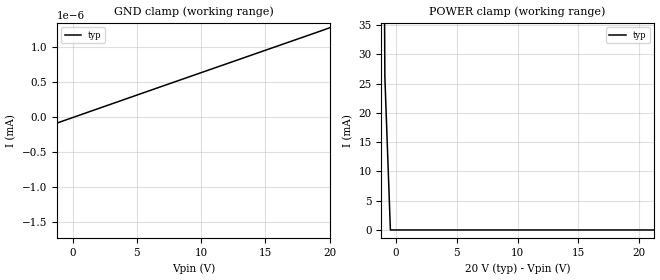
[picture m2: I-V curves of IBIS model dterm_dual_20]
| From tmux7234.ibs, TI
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| dterm_dual_20
[Model]   dterm_dual_20
Model_type   Terminator
|   typ   min   max
C_comp   1.598234e-11   NA   NA
[Voltage Range]   20   NA   NA
[Temperature Range]   27   NA   NA
[Power Clamp Reference]   20   NA   NA
[GND Clamp Reference]   0   NA   NA
[GND Clamp]
|   Voltage   I(typ)   I(min)   I(max)
-25V      -2.386A    NA         NA
-20.45V   -755.1nA   NA         NA
-20V      -1.317nA   NA         NA
-4.091V   -271.4pA   NA         NA
20V       1.28nA     NA         NA
[POWER Clamp]
|   Voltage   I(typ)   I(min)   I(max)
-5V       3.082A     NA         NA
-1.364V   208.9mA    NA         NA
-909.1mV  26.14mA    NA         NA
-454.5mV  952.4nA    NA         NA
40V       -1.317nA   NA         NA
